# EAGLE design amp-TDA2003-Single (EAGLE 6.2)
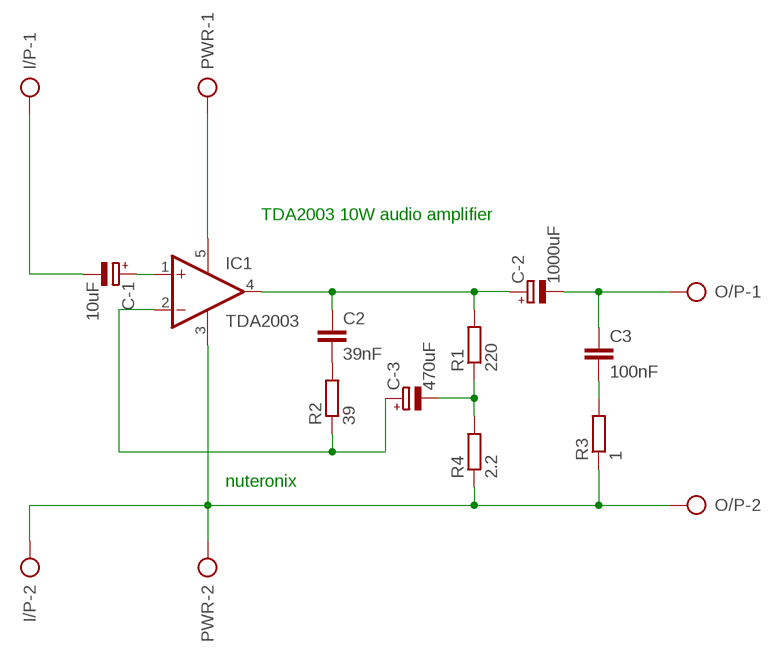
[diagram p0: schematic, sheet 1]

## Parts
C2  39nF  C-EU050-025X075  [C050-025X075]
C3  100nF  C-EU050-025X075  [C050-025X075]
C-1  10uF  CPOL-EUE5-6  [E5-6]
C-2  1000uF  CPOL-EUE5-8.5  [E5-8,5]
C-3  470uF  CPOL-EUE5-8.5  [E5-8,5]
I/P  AK500/2  [AK500/2]
IC1  TDA2003  TDA2030V  [CB360]
O/P  AK500/2  [AK500/2]
PWR  AK500/2  [AK500/2]
R1  220  R-EU_0207/7  [0207/7]
R2  39  R-EU_0207/7  [0207/7]
R3  1  R-EU_0207/7  [0207/7]
R4  2.2  R-EU_0207/7  [0207/7]

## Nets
N$1: C-1.- I/P.1
N$3: C3.2 R3.2
N$4: C-1.+ IC1.1(+IN)
N$5: C2.2 R2.2
N$6: C2.1 C-2.+ IC1.4(OUT) R1.2
N$7: C-3.+ IC1.2(-IN) R2.1
N$8: C-3.- R1.1 R4.2
N$9: I/P.2 IC1.3(GND) O/P.2 PWR.2 R3.1 R4.1
N$10: IC1.5(V+) PWR.1
N$14: C3.1 C-2.- O/P.1

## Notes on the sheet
- TDA2003 10W audio amplifier
- nuteronix

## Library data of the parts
C2 C3 = rcl:C-EU: CAPACITOR, European symbol
C-1-C-3 = rcl:CPOL-EU: POLARIZED CAPACITOR, European symbol
I/P O/P PWR = con-ptr500:AK500/2: CONNECTOR
IC1 = linear:TDA2030: Power OP AMP
R1-R4 = resistor:R-EU_: RESISTOR, European symbol

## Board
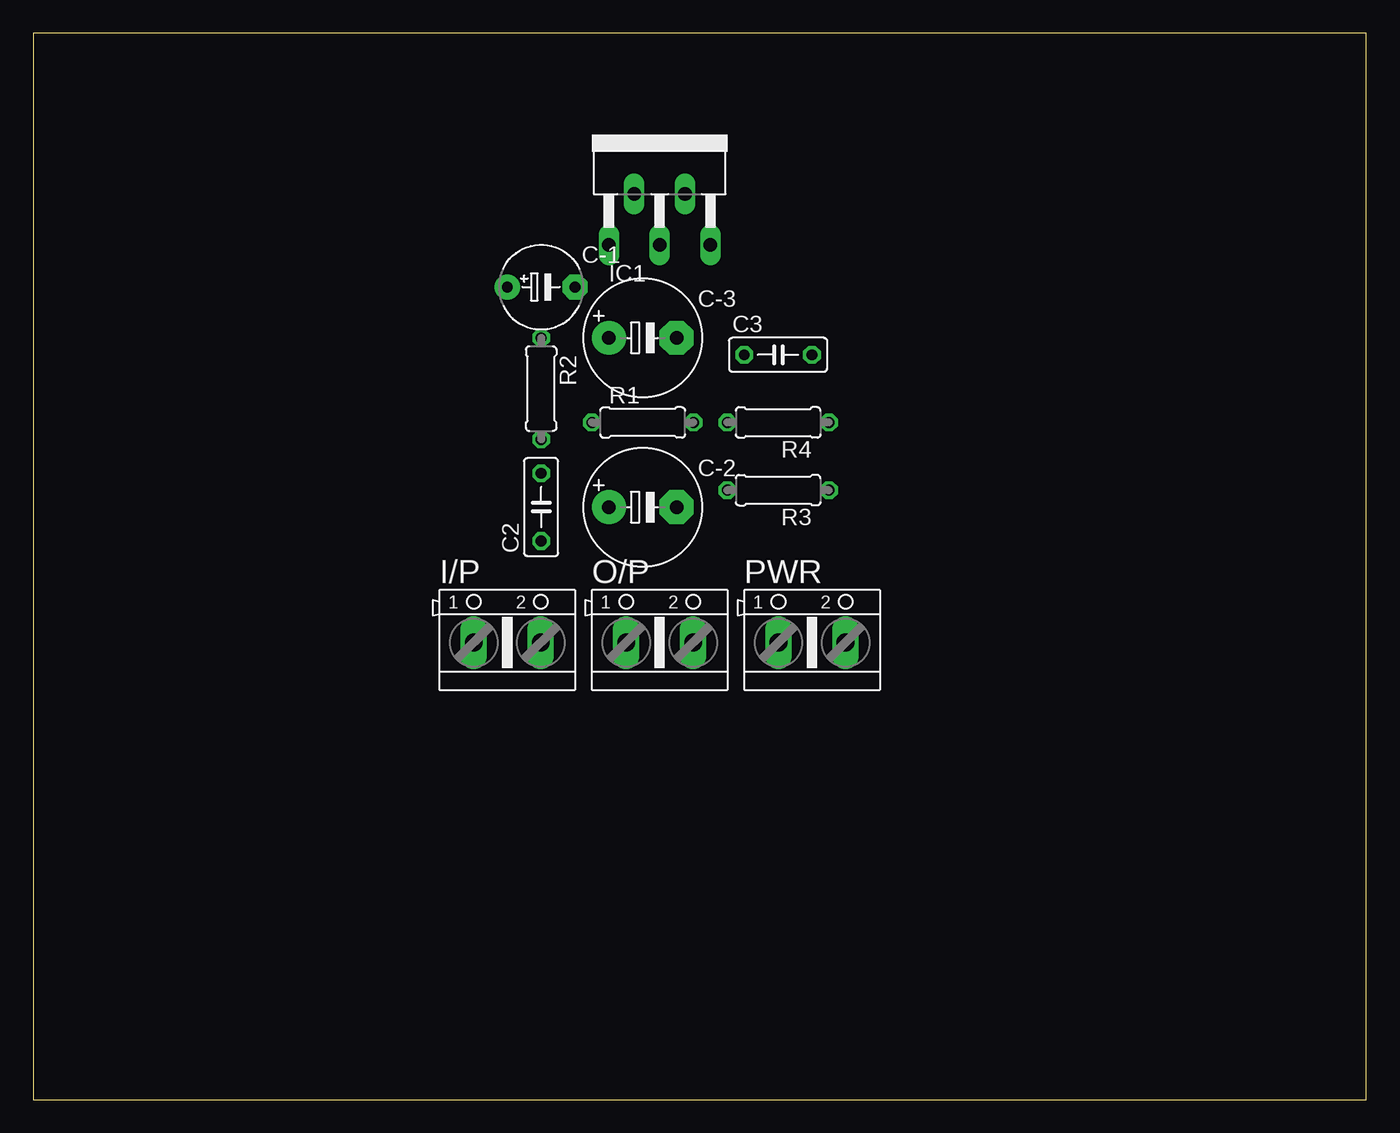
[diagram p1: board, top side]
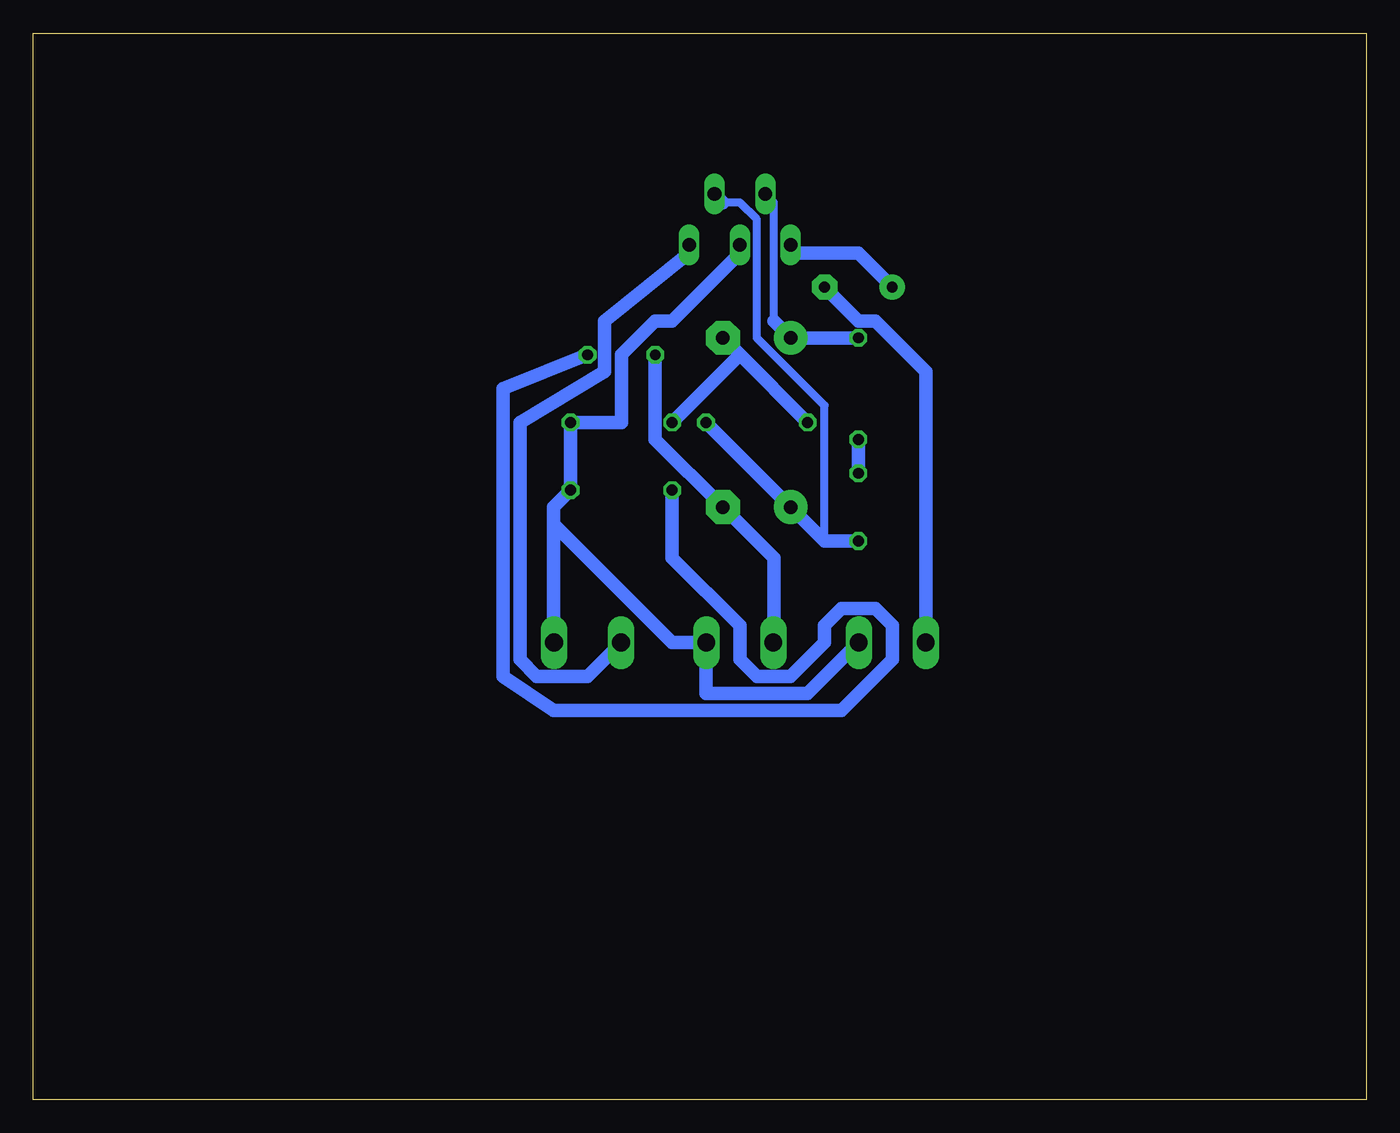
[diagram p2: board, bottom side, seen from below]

Size 100 x 80 mm. Coordinates in mm from the lower left corner, seen from the top.
Outline: 0,0 100,0 100,80 0,80 0,0
Copper layers (1*16): Top 0.035mm / dielectric 1.5mm / Bottom 0.035mm
Design rules: minimum track width 10mil, minimum drill 24mil, track to track 8mil, track to pad 8mil, pad to pad 8mil, via to via 8mil, smd to smd 8mil, copper to edge 40mil, drill to drill 8mil, minimum pad ring 10mil, minimum via ring 8mil, stop-mask expansion 4mil, vias tented up to drill 0mil, thermal gap 10mil

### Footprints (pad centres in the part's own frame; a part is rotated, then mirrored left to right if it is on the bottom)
C050-025X075 = drill 0.813 octagon: 1 -2.54,0; 2 2.54,0
E5-6 = drill 0.813 pad 1.905: + -2.54,0 | drill 0.813 pad 1.905 octagon: - 2.54,0
E5-8,5 = drill 1.016 pad 2.54: + -2.54,0 | drill 1.016 pad 2.54 octagon: - 2.54,0
AK500/2 = drill 1.321 long: 1 -2.515,0; 2 2.515,0
CB360 = drill 1.016 long: 1 -3.81,-8.255; 2 -1.905,-4.445; 3 0,-8.255; 4 1.905,-4.445; 5 3.81,-8.255
0207/7 = drill 0.813 octagon: 1 -3.81,0; 2 3.81,0

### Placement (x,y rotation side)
C2  38.1,44.45 90 top
C3  55.88,55.88 0 top
C-1  38.1,60.96 0 top
C-2  45.72,44.45 0 top
C-3  45.72,57.15 0 top
I/P  35.56,34.29 0 top
IC1  46.99,72.39 0 top
O/P  46.99,34.29 0 top
PWR  58.42,34.29 0 top
R1  45.72,50.8 0 top
R2  38.1,53.34 270 top
R3  55.88,45.72 180 top
R4  55.88,50.8 180 top

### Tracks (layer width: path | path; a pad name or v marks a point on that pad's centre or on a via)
N$1
  Bottom 1.016: C-1.- 38.1,58.42 36.83,58.42 33.02,54.61 33.02,34.29 I/P.1
N$3
  Bottom 1.016: R3.2 52.07,40.64 46.99,35.56 46.99,33.02 45.72,31.75 43.18,31.75 40.64,34.29 40.64,35.56 39.37,36.83 36.83,36.83 35.56,35.56 35.56,33.02 39.37,29.21 60.96,29.21 64.77,31.75 64.77,53.34 C3.2
N$4
  Bottom 1.016: C-1.+ 38.1,63.5 43.18,63.5 IC1.1
N$5
  Bottom 1.016: R2.2 C2.2
N$6
  Bottom 0.61: 48.26,67.31 46.99,67.31 45.72,66.04 45.72,57.15 40.64,52.07 40.64,41.91
  Bottom 1.016: C2.1 40.64,41.91 C-2.+ R1.2 | 48.26,67.31 IC1.4
N$7
  Bottom 0.61: 44.45,58.42 44.45,67.31 IC1.2
  Bottom 1.016: R2.1 C-3.+ 44.45,58.42
N$8
  Bottom 1.016: C-3.- 46.99,55.88 | 46.99,55.88 R1.1 | 46.99,55.88 R4.2
N$9
  Bottom 1.016: 49.53,34.29 49.53,30.48 41.91,30.48 38.1,34.29 I/P.2 | IC1.3 46.99,63.5 52.07,58.42 53.34,58.42 55.88,55.88 55.88,50.8 R4.1 R3.1 60.96,44.45 60.96,43.18 | 60.96,43.18 60.96,34.29 PWR.2 | 49.53,34.29 52.07,34.29 60.96,43.18 | 49.53,34.29 O/P.2
N$10
  Bottom 1.016: IC1.5 50.8,63.5 57.15,58.42 57.15,54.61 63.5,50.8 63.5,33.02 62.23,31.75 58.42,31.75 55.88,34.29 PWR.1
N$14
  Bottom 1.016: C3.1 53.34,49.53 C-2.- 44.45,40.64 44.45,34.29 O/P.1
